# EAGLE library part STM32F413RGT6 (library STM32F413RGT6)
ARM Microcontrollers - MCU High-performance access line, ARM Cortex-M4 core with DSP and FPU, 1 MByte Flash, 100 MHz CPU, ART Accelerator Source: Datasheet
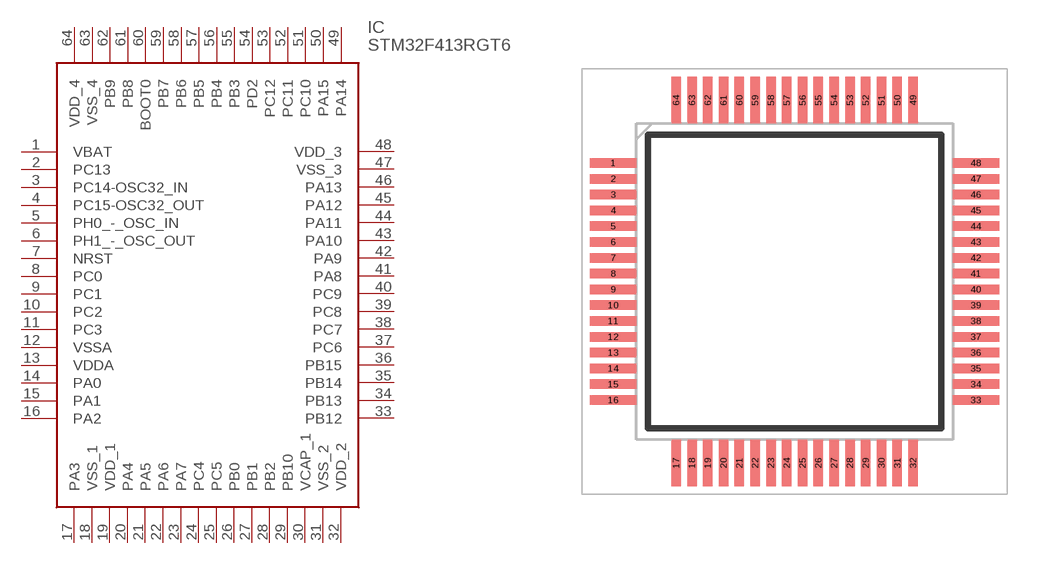
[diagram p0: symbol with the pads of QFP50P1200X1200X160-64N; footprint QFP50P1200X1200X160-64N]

Designator prefix IC

## STM32F413RGT6 (Description: ARM Microcontrollers - MCU High-performance access line, ARM Cortex-M4 core with DSP and FPU, 1 MByte Flash, 100 MHz CPU, ART Accelerator; Height: 1.6mm; Manufacturer_Name: STMicroelectronics; Manufacturer_Part_Number: STM32F413RGT6; Mouser_Part_Number: 511-STM32F413RGT6; Mouser_Price-Stock: https://www.mouser.co.uk/ProductDetail/STMicroelectronics/STM32F413RGT6?qs=FNcb6ahWXRyREY%252BFzgYY7A%3D%3D)  [QFP50P1200X1200X160-64N]
1  VBAT
2  PC13
3  PC14-OSC32_IN
4  PC15-OSC32_OUT
5  PH0_-_OSC_IN
6  PH1_-_OSC_OUT
7  NRST
8  PC0
9  PC1
10  PC2
11  PC3
12  VSSA
13  VDDA
14  PA0
15  PA1
16  PA2
17  PA3
18  VSS_1
19  VDD_1
20  PA4
21  PA5
22  PA6
23  PA7
24  PC4
25  PC5
26  PB0
27  PB1
28  PB2
29  PB10
30  VCAP_1
31  VSS_2
32  VDD_2
33  PB12
34  PB13
35  PB14
36  PB15
37  PC6
38  PC7
39  PC8
40  PC9
41  PA8
42  PA9
43  PA10
44  PA11
45  PA12
46  PA13
47  VSS_3
48  VDD_3
49  PA14
50  PA15
51  PC10
52  PC11
53  PC12
54  PD2
55  PB3
56  PB4
57  PB5
58  PB6
59  PB7
60  BOOT0
61  PB8
62  PB9
63  VSS_4
64  VDD_4

## Footprint QFP50P1200X1200X160-64N (pad centres in mm)
LQFP, 10 X 10 X 1.4 PKG, 0.5 PITCH, 64LD
smd 1.475 x 0.3: 1 -5.738,3.75; 2 -5.738,3.25; 3 -5.738,2.75; 4 -5.738,2.25; 5 -5.738,1.75; 6 -5.738,1.25; 7 -5.738,0.75; 8 -5.738,0.25; 9 -5.738,-0.25; 10 -5.738,-0.75; 11 -5.738,-1.25; 12 -5.738,-1.75; 13 -5.738,-2.25; 14 -5.738,-2.75; 15 -5.738,-3.25; 16 -5.738,-3.75; 33 5.738,-3.75; 34 5.738,-3.25; 35 5.738,-2.75; 36 5.738,-2.25; 37 5.738,-1.75; 38 5.738,-1.25; 39 5.738,-0.75; 40 5.738,-0.25; 41 5.738,0.25; 42 5.738,0.75; 43 5.738,1.25; 44 5.738,1.75; 45 5.738,2.25; 46 5.738,2.75; 47 5.738,3.25; 48 5.738,3.75
smd 0.3 x 1.475: 17 -3.75,-5.738; 18 -3.25,-5.738; 19 -2.75,-5.738; 20 -2.25,-5.738; 21 -1.75,-5.738; 22 -1.25,-5.738; 23 -0.75,-5.738; 24 -0.25,-5.738; 25 0.25,-5.738; 26 0.75,-5.738; 27 1.25,-5.738; 28 1.75,-5.738; 29 2.25,-5.738; 30 2.75,-5.738; 31 3.25,-5.738; 32 3.75,-5.738; 49 3.75,5.738; 50 3.25,5.738; 51 2.75,5.738; 52 2.25,5.738; 53 1.75,5.738; 54 1.25,5.738; 55 0.75,5.738; 56 0.25,5.738; 57 -0.25,5.738; 58 -0.75,5.738; 59 -1.25,5.738; 60 -1.75,5.738; 61 -2.25,5.738; 62 -2.75,5.738; 63 -3.25,5.738; 64 -3.75,5.738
